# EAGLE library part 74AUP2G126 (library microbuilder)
74AUP2G126 - Low-Power Dual Tri-State Buffer OE high enables output. For OE Low enabled output use 74AUP2G125. VCC: 0.8-3.6V Temp: -40°C - 125°C Package Variant: 8-VSSOP (SOT765-1) Manuf. ID: 74AUP2G126DC,125 Digikey: 568-4987-1-ND NOTE: Make sure to check the propogation delay to see if it's short enough for your timing since it's largely dependant on the line capacitance and supply voltage!
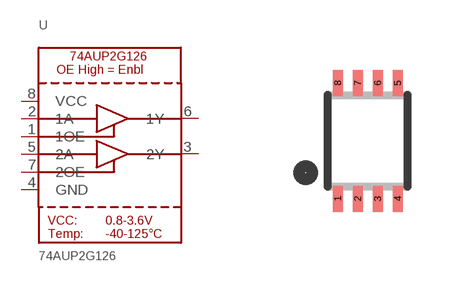
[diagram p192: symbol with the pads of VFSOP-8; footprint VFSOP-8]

Designator prefix U

## 74AUP2G126  [VFSOP-8]
1  1OE  in
2  1A  in
3  2Y  out
4  GND  pwr
5  2A  in
6  1Y  out
7  2OE  in
8  VCC  pwr

## Footprint VFSOP-8 (pad centres in mm)
VFSOP8 - 0.5mm pitch, 2.0x2.3mm Source: http://focus.ti.com/lit/ds/symlink/txs0102.pdf
smd 0.25 x 0.65: 1 -0.75,-1.45; 2 -0.25,-1.45; 3 0.25,-1.45; 4 0.75,-1.45; 5 0.75,1.45; 6 0.25,1.45; 7 -0.25,1.45; 8 -0.75,1.45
